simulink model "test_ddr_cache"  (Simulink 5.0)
settings: Solver=ode45  StartTime=0.0  StopTime=10.0  RelTol=1e-3
undefined symbols (not defined in the file or in its folder): Bit, Location, Lower, tmp20, Width
libraries: xbsIndex_r3 x61, ADlibrary x2

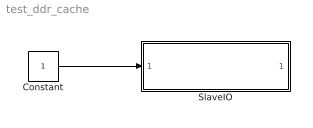
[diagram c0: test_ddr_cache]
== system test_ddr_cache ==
  Constant : Constant
  SlaveIO : Subsystem
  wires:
  Constant/1 -> SlaveIO/1(Vector Input)

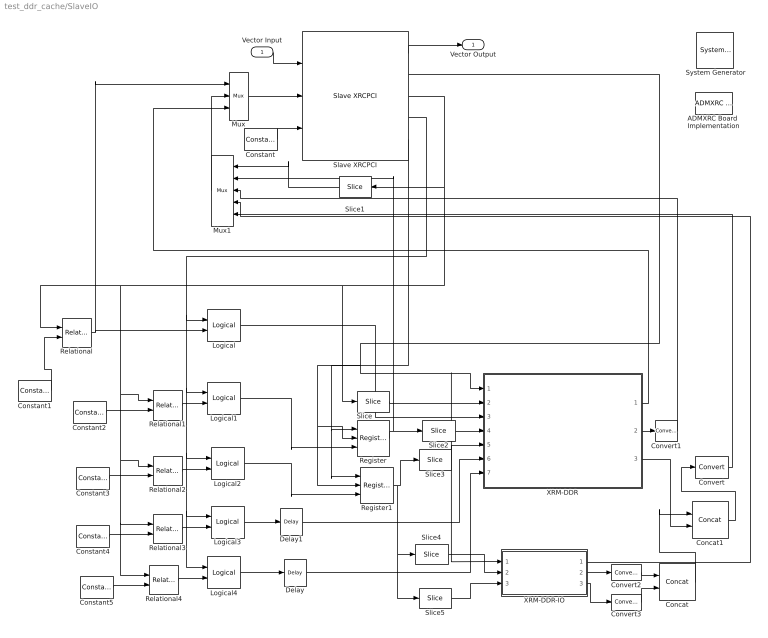
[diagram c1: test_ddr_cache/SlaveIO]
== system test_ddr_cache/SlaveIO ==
  Vector Input : Inport
  " System Generator" : xbsIndex_r3/ System Generator  Tag=genX  xilinxfamily=Virtex2  part=xc2v6000  speed=-4  package=ff1152  synthesis_tool=XST  directory=e:/tmp20  testbench=off  simulink_period=1  sysclk_period=9  incr_netlist=off  trim_vbits=According to Block Masks  dbl_ovrd=According to Block Masks  core_generation=According to Block Masks  run_coregen=off  deprecated_control=off  eval_field=0
  ADMXRC Board  Implementation : ADlibrary/Miscellaneous/ADMXRC Board  Implementation  board=XRCII  run_synth=on  make_clean=off  userdefmods=ddr_cache.txt xrmddrio.txt  lvds_io_std=3.3v  clock_source=MCLK
  Concat : xbsIndex_r3/Concat  num_inputs=2  explicit_period=off  period=1  dbl_ovrd=off
  Concat1 : xbsIndex_r3/Concat  num_inputs=2  explicit_period=off  period=1  dbl_ovrd=off
  Constant : xbsIndex_r3/Constant  const=1  arith_type=Unsigned  n_bits=1  bin_pt=0  explicit_period=on  period=1  dbl_ovrd=off
  Constant1 : xbsIndex_r3/Constant  const=2047  arith_type=Unsigned  n_bits=22  bin_pt=0  explicit_period=off  period=1  dbl_ovrd=off
  Constant2 : xbsIndex_r3/Constant  const=0  arith_type=Unsigned  n_bits=22  bin_pt=0  explicit_period=off  period=1  dbl_ovrd=off
  Constant3 : xbsIndex_r3/Constant  const=4  arith_type=Unsigned  n_bits=22  bin_pt=0  explicit_period=off  period=1  dbl_ovrd=off
  Constant4 : xbsIndex_r3/Constant  const=8  arith_type=Unsigned  n_bits=22  bin_pt=0  explicit_period=off  period=1  dbl_ovrd=off
  Constant5 : xbsIndex_r3/Constant  const=12  arith_type=Unsigned  n_bits=22  bin_pt=0  explicit_period=off  period=1  dbl_ovrd=off
  Convert : xbsIndex_r3/Convert  arith_type=Unsigned  n_bits=32  bin_pt=0  quantization=Truncate  overflow=Wrap  latency=0  explicit_period=off  period=1  dbl_ovrd=off  inserted_by_tool=off
  Convert1 : xbsIndex_r3/Convert  arith_type=Unsigned  n_bits=32  bin_pt=0  quantization=Truncate  overflow=Wrap  latency=0  explicit_period=off  period=1  dbl_ovrd=off  inserted_by_tool=off
  Convert2 : xbsIndex_r3/Convert  arith_type=Unsigned  n_bits=1  bin_pt=0  quantization=Truncate  overflow=Wrap  latency=0  explicit_period=off  period=1  dbl_ovrd=off  inserted_by_tool=off
  Convert3 : xbsIndex_r3/Convert  arith_type=Unsigned  n_bits=1  bin_pt=0  quantization=Truncate  overflow=Wrap  latency=0  explicit_period=off  period=1  dbl_ovrd=off  inserted_by_tool=off
  Delay : xbsIndex_r3/Delay  latency=1  reg_retiming=off  explicit_period=off  period=1  en=off  accept_only_valid=off  init_zero=on  dbl_ovrd=off
  Delay1 : xbsIndex_r3/Delay  latency=1  reg_retiming=off  explicit_period=off  period=1  en=off  accept_only_valid=off  init_zero=on  dbl_ovrd=off
  Logical{,1..4} (5 alike) : xbsIndex_r3/Logical  logical_function=AND  inputs=2  precision=Full  arith_type=Unsigned  n_bits=8  bin_pt=2  align_bp=on  latency=0  explicit_period=off  period=1  en=off  dbl_ovrd=off
  Mux : xbsIndex_r3/Mux  inputs=2  precision=Full  arith_type="Signed  (2's comp)"  n_bits=8  bin_pt=2  quantization=Truncate  overflow=Wrap  latency=0  mux_type=off  explicit_period=off  period=1  en=off  dbl_ovrd=off  use_rpm=off  gen_core=on
  Mux1 : xbsIndex_r3/Mux  Orientation=left  inputs=4  precision=Full  arith_type="Signed  (2's comp)"  n_bits=8  bin_pt=2  quantization=Truncate  overflow=Wrap  latency=0  mux_type=off  explicit_period=off  period=1  en=off  dbl_ovrd=off  use_rpm=off  gen_core=on
  Register : xbsIndex_r3/Register  init=0  reg_only_valid=off  explicit_period=off  period=1  rst=on  en=on  out_en=off  dbl_ovrd=off
  Register1 : xbsIndex_r3/Register  init=0  reg_only_valid=off  explicit_period=off  period=1  rst=on  en=on  out_en=off  dbl_ovrd=off
  Relational : xbsIndex_r3/Relational  mode=a>b  latency=0  explicit_period=off  period=1  en=off  dbl_ovrd=off
  Relational{1..4} (4 alike) : xbsIndex_r3/Relational  mode=a=b  latency=0  explicit_period=off  period=1  en=off  dbl_ovrd=off
  Slave XRCPCI : ADlibrary/PCI/Slave XRCPCI  no_inputs=1  no_outputs=1  circuit_lag=1  decode_delay=0
  Slice : xbsIndex_r3/Slice  mode=Lower Bit Location + Width  nbits=11  bit1=0  base1=MSB of Input  bit0=0  base0=LSB of Input  boolean_output=off  explicit_period=off  period=1  dbl_ovrd=off
  Slice1 : xbsIndex_r3/Slice  Orientation=left  mode=Lower Bit Location + Width  nbits=2  bit1=0  base1=MSB of Input  bit0=0  base0=LSB of Input  boolean_output=off  explicit_period=off  period=1  dbl_ovrd=off
  Slice2 : xbsIndex_r3/Slice  mode=Lower Bit Location + Width  nbits=16  bit1=0  base1=MSB of Input  bit0=0  base0=LSB of Input  boolean_output=off  explicit_period=off  period=1  dbl_ovrd=off
  Slice3 : xbsIndex_r3/Slice  mode=Lower Bit Location + Width  nbits=7  bit1=0  base1=MSB of Input  bit0=0  base0=LSB of Input  boolean_output=off  explicit_period=off  period=1  dbl_ovrd=off
  Slice4 : xbsIndex_r3/Slice  mode=Lower Bit Location + Width  nbits=1  bit1=0  base1=MSB of Input  bit0=8  base0=LSB of Input  boolean_output=off  explicit_period=off  period=1  dbl_ovrd=off
  Slice5 : xbsIndex_r3/Slice  mode=Lower Bit Location + Width  nbits=1  bit1=0  base1=MSB of Input  bit0=8  base0=LSB of Input  boolean_output=off  explicit_period=off  period=1  dbl_ovrd=off
  XRM-DDR : Subsystem
  XRM-DDR-IO : Subsystem
  Vector Output : Outport
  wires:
  Slave XRCPCI/1 -> Vector Output/1
  Vector Input/1 -> Slave XRCPCI/1
  Slave XRCPCI/2 -> Register/1, Register1/1, XRM-DDR/1(c_data_in), XRM-DDR-IO/1(data_out)
  Constant/1 -> Slave XRCPCI/3
  Slave XRCPCI/3 -> Slice/1, Relational/1, Relational4/1, Relational3/1, Relational2/1, Relational1/1, Slice1/1
  Slave XRCPCI/4 -> Logical/1, Logical1/1, Logical2/1, Logical3/1, Logical4/1
  Relational/1 -> Logical/2, Mux/1
  Logical/1 -> XRM-DDR/3(c_write)
  Slice/1 -> XRM-DDR/2(c_addr)
  Constant1/1 -> Relational/2
  Constant2/1 -> Relational1/2
  Mux/1 -> Slave XRCPCI/2
  XRM-DDR/1(c_data_out) -> Mux/3
  Slice1/1 -> Mux1/1
  Mux1/1 -> Mux/2
  Slice2/1 -> XRM-DDR/4(page)
  Slice3/1 -> XRM-DDR/5(addr)
  Register/1 -> Slice2/1, Mux1/2
  Slave XRCPCI/5 -> Register/2, Register1/2
  Register1/1 -> Slice3/1, Slice5/1, Slice4/1
  Relational1/1 -> Logical1/2
  Constant3/1 -> Relational2/2
  Relational2/1 -> Logical2/2
  Constant4/1 -> Relational3/2
  Relational3/1 -> Logical3/2
  Constant5/1 -> Relational4/2
  Relational4/1 -> Logical4/2
  Logical1/1 -> Register/3
  Logical2/1 -> Register1/3
  Logical3/1 -> Delay1/1
  Logical4/1 -> Delay/1
  XRM-DDR/2(busy) -> Convert1/1
  Convert/1 -> Mux1/5
  Convert1/1 -> Mux1/3
  Delay/1 -> XRM-DDR/7(write)
  Delay1/1 -> XRM-DDR/6(read)
  XRM-DDR-IO/1(data_in) -> Mux1/4
  Slice5/1 -> XRM-DDR-IO/3(read)
  Slice4/1 -> XRM-DDR-IO/2(dir)
  Concat/1 -> Concat1/1
  Concat1/1 -> Convert/1
  Convert2/1 -> Concat/1
  Convert3/1 -> Concat/2
  XRM-DDR-IO/3(full) -> Convert3/1
  XRM-DDR-IO/2(empty) -> Convert2/1
  XRM-DDR/3(status) -> Concat1/2

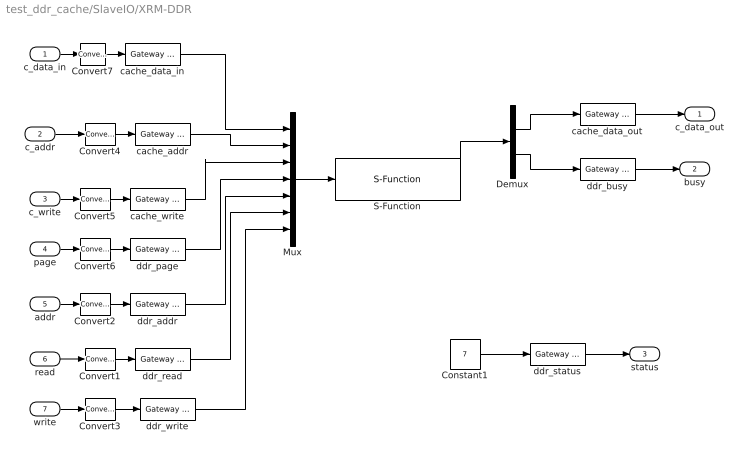
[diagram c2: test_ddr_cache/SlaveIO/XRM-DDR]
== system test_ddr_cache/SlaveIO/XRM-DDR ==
  c_data_in : Inport
  c_addr : Inport  Port=2
  c_write : Inport  Port=3
  page : Inport  Port=4
  addr : Inport  Port=5
  read : Inport  Port=6
  write : Inport  Port=7
  Constant1 : Constant  Value=7
  Convert1 : xbsIndex_r3/Convert  arith_type=Boolean  n_bits=8  bin_pt=6  quantization=Truncate  overflow=Wrap  latency=0  explicit_period=on  period=1  dbl_ovrd=off  inserted_by_tool=off
  Convert2 : xbsIndex_r3/Convert  arith_type=Unsigned  n_bits=7  bin_pt=0  quantization=Truncate  overflow=Wrap  latency=0  explicit_period=on  period=1  dbl_ovrd=off  inserted_by_tool=off
  Convert3 : xbsIndex_r3/Convert  arith_type=Boolean  n_bits=8  bin_pt=6  quantization=Truncate  overflow=Wrap  latency=0  explicit_period=on  period=1  dbl_ovrd=off  inserted_by_tool=off
  Convert4 : xbsIndex_r3/Convert  arith_type=Unsigned  n_bits=11  bin_pt=0  quantization=Truncate  overflow=Wrap  latency=0  explicit_period=on  period=1  dbl_ovrd=off  inserted_by_tool=off
  Convert5 : xbsIndex_r3/Convert  arith_type=Boolean  n_bits=25  bin_pt=0  quantization=Truncate  overflow=Wrap  latency=0  explicit_period=on  period=1  dbl_ovrd=off  inserted_by_tool=off
  Convert6 : xbsIndex_r3/Convert  arith_type=Unsigned  n_bits=16  bin_pt=0  quantization=Truncate  overflow=Wrap  latency=0  explicit_period=on  period=1  dbl_ovrd=off  inserted_by_tool=off
  Convert7 : xbsIndex_r3/Convert  arith_type=Unsigned  n_bits=32  bin_pt=0  quantization=Truncate  overflow=Wrap  latency=0  explicit_period=on  period=1  dbl_ovrd=off  inserted_by_tool=off
  Demux : Demux  Outputs=2
  Mux : Mux  Inputs=7
  S-Function : S-Function  FunctionName=model_ddrram_cache
  cache_addr : xbsIndex_r3/Gateway Out  hdl_port=on  timing_constraint=None  locs_specified=off  LOCs={}  needs_fixed_name=on
  cache_data_in : xbsIndex_r3/Gateway Out  hdl_port=on  timing_constraint=None  locs_specified=off  LOCs={}  needs_fixed_name=on
  cache_data_out : xbsIndex_r3/Gateway In  arith_type=Unsigned  n_bits=32  bin_pt=0  quantization=Truncate  overflow=Wrap  period=1  timing_constraint=None  locs_specified=off  LOCs={}  needs_fixed_name=on  dbl_ovrd=off
  cache_write : xbsIndex_r3/Gateway Out  hdl_port=on  timing_constraint=None  locs_specified=off  LOCs={}  needs_fixed_name=on
  ddr_addr : xbsIndex_r3/Gateway Out  hdl_port=on  timing_constraint=None  locs_specified=off  LOCs={}  needs_fixed_name=on
  ddr_busy : xbsIndex_r3/Gateway In  arith_type=Boolean  n_bits=1  bin_pt=0  quantization=Truncate  overflow=Wrap  period=1  timing_constraint=None  locs_specified=off  LOCs={}  needs_fixed_name=on  dbl_ovrd=off
  ddr_page : xbsIndex_r3/Gateway Out  hdl_port=on  timing_constraint=None  locs_specified=off  LOCs={}  needs_fixed_name=on
  ddr_read : xbsIndex_r3/Gateway Out  hdl_port=on  timing_constraint=None  locs_specified=off  LOCs={}  needs_fixed_name=on
  ddr_status : xbsIndex_r3/Gateway In  arith_type=Unsigned  n_bits=3  bin_pt=0  quantization=Truncate  overflow=Wrap  period=1  timing_constraint=None  locs_specified=off  LOCs={}  needs_fixed_name=on  dbl_ovrd=off
  ddr_write : xbsIndex_r3/Gateway Out  hdl_port=on  timing_constraint=None  locs_specified=off  LOCs={}  needs_fixed_name=on
  c_data_out : Outport
  busy : Outport  Port=2
  status : Outport  Port=3
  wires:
  c_data_in/1 -> Convert7/1
  addr/1 -> Convert2/1
  write/1 -> Convert3/1
  read/1 -> Convert1/1
  cache_data_out/1 -> c_data_out/1
  ddr_busy/1 -> busy/1
  Convert3/1 -> ddr_write/1
  Convert1/1 -> ddr_read/1
  Constant1/1 -> ddr_status/1
  ddr_status/1 -> status/1
  Convert2/1 -> ddr_addr/1
  Convert7/1 -> cache_data_in/1
  c_addr/1 -> Convert4/1
  Convert4/1 -> cache_addr/1
  c_write/1 -> Convert5/1
  Convert5/1 -> cache_write/1
  page/1 -> Convert6/1
  Convert6/1 -> ddr_page/1
  Demux/1 -> cache_data_out/1
  Demux/2 -> ddr_busy/1
  cache_data_in/1 -> Mux/1
  cache_addr/1 -> Mux/2
  cache_write/1 -> Mux/3
  ddr_page/1 -> Mux/4
  ddr_addr/1 -> Mux/5
  ddr_read/1 -> Mux/6
  ddr_write/1 -> Mux/7
  Mux/1 -> S-Function/1
  S-Function/1 -> Demux/1

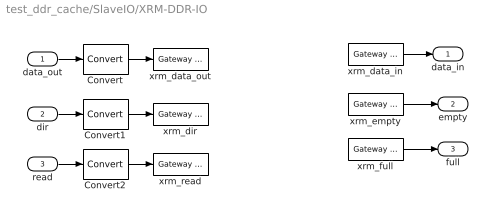
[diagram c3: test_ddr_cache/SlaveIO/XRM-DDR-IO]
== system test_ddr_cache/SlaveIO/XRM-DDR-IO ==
  data_out : Inport
  dir : Inport  Port=2
  read : Inport  Port=3
  Convert : xbsIndex_r3/Convert  arith_type=Unsigned  n_bits=32  bin_pt=0  quantization=Truncate  overflow=Wrap  latency=0  explicit_period=off  period=1  dbl_ovrd=off  inserted_by_tool=off
  Convert1 : xbsIndex_r3/Convert  arith_type=Boolean  n_bits=32  bin_pt=0  quantization=Truncate  overflow=Wrap  latency=0  explicit_period=off  period=1  dbl_ovrd=off  inserted_by_tool=off
  Convert2 : xbsIndex_r3/Convert  arith_type=Boolean  n_bits=32  bin_pt=0  quantization=Truncate  overflow=Wrap  latency=0  explicit_period=off  period=1  dbl_ovrd=off  inserted_by_tool=off
  xrm_data_in : xbsIndex_r3/Gateway In  arith_type=Unsigned  n_bits=32  bin_pt=0  quantization=Truncate  overflow=Wrap  period=1  timing_constraint=None  locs_specified=off  LOCs={}  needs_fixed_name=on  dbl_ovrd=off
  xrm_data_out : xbsIndex_r3/Gateway Out  hdl_port=on  timing_constraint=None  locs_specified=off  LOCs={}  needs_fixed_name=on
  xrm_dir : xbsIndex_r3/Gateway Out  hdl_port=on  timing_constraint=None  locs_specified=off  LOCs={}  needs_fixed_name=on
  xrm_empty : xbsIndex_r3/Gateway In  arith_type=Boolean  n_bits=8  bin_pt=6  quantization=Truncate  overflow=Wrap  period=1  timing_constraint=None  locs_specified=off  LOCs={}  needs_fixed_name=on  dbl_ovrd=off
  xrm_full : xbsIndex_r3/Gateway In  arith_type=Boolean  n_bits=8  bin_pt=6  quantization=Truncate  overflow=Wrap  period=1  timing_constraint=None  locs_specified=off  LOCs={}  needs_fixed_name=on  dbl_ovrd=off
  xrm_read : xbsIndex_r3/Gateway Out  hdl_port=on  timing_constraint=None  locs_specified=off  LOCs={}  needs_fixed_name=on
  data_in : Outport
  empty : Outport  Port=2
  full : Outport  Port=3
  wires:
  xrm_data_in/1 -> data_in/1
  xrm_empty/1 -> empty/1
  xrm_full/1 -> full/1
  read/1 -> Convert2/1
  dir/1 -> Convert1/1
  data_out/1 -> Convert/1
  Convert/1 -> xrm_data_out/1
  Convert1/1 -> xrm_dir/1
  Convert2/1 -> xrm_read/1
